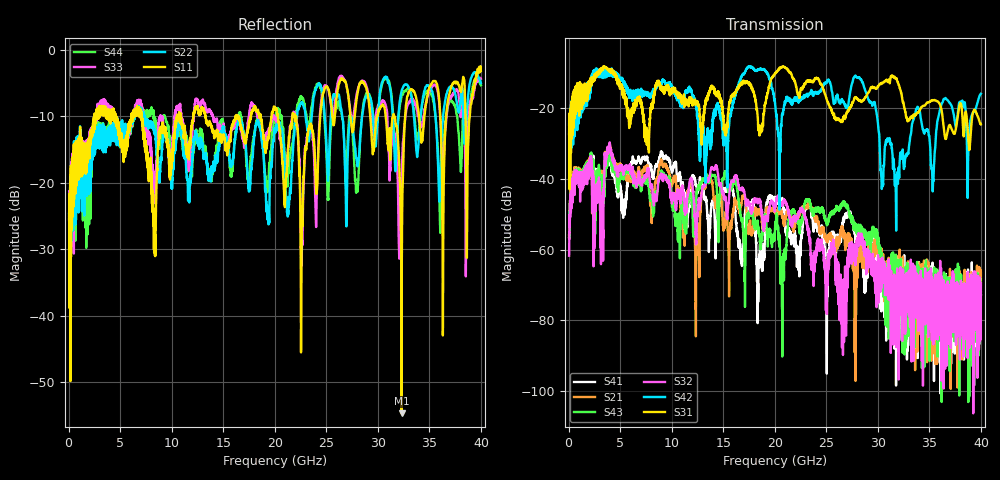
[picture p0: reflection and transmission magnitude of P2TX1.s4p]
!Agilent Technologies,N5245A,MY49151084,A.09.20.08
!Agilent N5245A: A.09.20.08
!Date: Thursday, March 01, 2012 14:32:21
!Correction: S11(Full 4 Port(1,2,3,4))
!S12(Full 4 Port(1,2,3,4))
!S13(Full 4 Port(1,2,3,4))
!S14(Full 4 Port(1,2,3,4))
!S21(Full 4 Port(1,2,3,4))
!S22(Full 4 Port(1,2,3,4))
!S23(Full 4 Port(1,2,3,4))
!S24(Full 4 Port(1,2,3,4))
!S31(Full 4 Port(1,2,3,4))
!S32(Full 4 Port(1,2,3,4))
!S33(Full 4 Port(1,2,3,4))
!S34(Full 4 Port(1,2,3,4))
!S41(Full 4 Port(1,2,3,4))
!S42(Full 4 Port(1,2,3,4))
!S43(Full 4 Port(1,2,3,4))
!S44(Full 4 Port(1,2,3,4))
!S4P File: Measurements: <S11,S12,S13,S14>,
!<S21,S22,S23,S24>,
!<S31,S32,S33,S34>,
!<S41,S42,S43,S44>:
# Hz S  dB  R 50
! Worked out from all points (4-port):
!   3996 points, 50 MHz to 40 GHz, reference 50 ohm
!   strongest paths, dB at 50 MHz, 10.04 GHz, 20.03 GHz, 30.02 GHz, 40 GHz:
!     S31: -27.3, -14.4, -10.0, -13.8, -24.5
!     S42: -24.5, -13.8, -18.7, -24.4, -15.9
!     S32: -61.7, -45.6, -48.5, -61.5, -69.5
!     S43: -56.3, -46.9, -54.2, -56.7, -72.0
!     S21: -55.6, -41.3, -49.4, -57.4, -66.5
!     S41: -56.7, -37.7, -46.4, -66.6, -72.6
!   lowest |S11| = -54.6 dB at 32.31 GHz (marker M1), VSWR 1.00, Z = 49.8 + j0.0564 ohm
!   |S11| at or under -10 dB: start of sweep to 2.508 GHz; 7.102 GHz to 10.54 GHz (3.434 GHz wide, 38.9 % of centre); 13.27 GHz to 16.18 GHz (2.909 GHz wide, 19.8 % of centre)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
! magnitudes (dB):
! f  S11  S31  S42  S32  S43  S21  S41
! 50 MHz  -25.4  -27.3  -24.5  -61.7  -56.3  -55.6  -56.7
! 8.99 GHz  -12.3  -14.1  -13.1  -39.0  -38.0  -34.7  -32.4
! 14.24 GHz  -12.4  -15.3  -22.1  -36.5  -39.4  -47.4  -58.9
! 20.71 GHz  -15.8  -8.3  -21.7  -47.1  -76.9  -50.7  -46.2
! 27.91 GHz  -7.8  -17.0  -11.1  -61.6  -54.7  -67.1  -54.5
! 32.31 GHz  -54.6  -16.1  -34.3  -75.9  -74.3  -68.1  -70.0
! 40 GHz  -3.2  -24.5  -15.9  -69.5  -72.0  -66.5  -72.6
